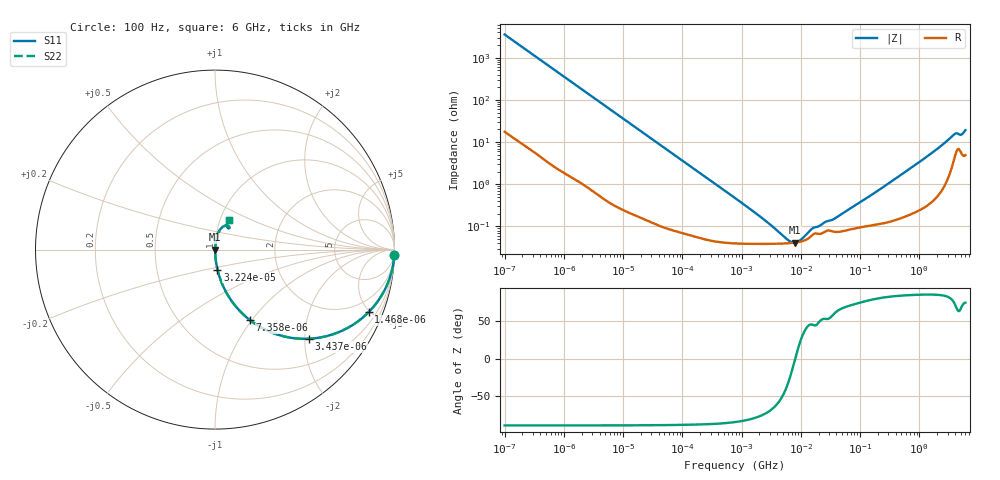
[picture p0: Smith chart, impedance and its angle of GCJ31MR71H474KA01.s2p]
!Murata Part Number: GCJ31MR71H474KA01
!These Parameters are Measured in Series Mode Connection
!Data Generated on Mar 13, 2026
!  o--ll--o
!Port1  Port2
!  o------o
!Operation Temp=25[degC], DC Bias Voltage=0[V]
!Freq. Start=100[Hz] Stop=6[GHz] 401[Steps]
# Hz S RI R 50
!Freq.(Hz) S11(Real) S11(Imag) S21(Real) S21(Imag) S12(Real) S12(Imag) S22(Real) S22(Imag)
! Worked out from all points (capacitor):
!   401 points, 100 Hz to 6 GHz, reference 50 ohm
!   read as one part in series: C = 447 nF near 109 Hz
!   lowest |Z| = 41.4 mohm at 7.948 MHz (marker M1)
!   series resonance near 8.045 MHz, so ESL is about 880 pH
!   S11 on the Smith chart (normalised r, x): 100 Hz: 1, -71; 1.468 kHz: 1.03, -4.89; 3.437 kHz: 1.01, -2.10; 7.358 kHz: 1.01, -0.98; 32.24 kHz: 1.00, -0.23; 6 GHz: 1.10, +0.37
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100  0.9991 -0.0281  0.000928 0.0281  0.000928 0.0281  0.9991 -0.0281
438  0.9846 -0.1206  0.0154 0.1206  0.0154 0.1206  0.9846 -0.1206
858  0.9448 -0.2259  0.0552 0.2259  0.0552 0.2259  0.9448 -0.2259
1468  0.8553 -0.349  0.1447 0.349  0.1447 0.349  0.8553 -0.349
2008  0.7607 -0.4238  0.2393 0.4238  0.2393 0.4238  0.7607 -0.4238
3437  0.5231 -0.4965  0.4769 0.4965  0.4769 0.4965  0.5231 -0.4965
7358  0.1954 -0.3934  0.8046 0.3934  0.8046 0.3934  0.1954 -0.3934
13772  0.0661 -0.2447  0.9339 0.2447  0.9339 0.2447  0.0661 -0.2447
32244  0.0137 -0.1109  0.9863 0.1109  0.9863 0.1109  0.0137 -0.1109
40335  0.00907 -0.0892  0.9909 0.0892  0.9909 0.0892  0.00907 -0.0892
774597  0.000418 -0.00471  0.9996 0.00471  0.9996 0.00471  0.000418 -0.00471
2372521  0.000388 -0.00142  0.9996 0.00142  0.9996 0.00142  0.000388 -0.00142
6075234  0.0004 -0.000263  0.9996 0.000263  0.9996 0.000263  0.0004 -0.000263
7947587  0.000414 -1.12e-05  0.9996 1.12e-05  0.9996 1.12e-05  0.000414 -1.12e-05
9941735  0.000437 0.000201  0.9996 -0.000201  0.9996 -0.000201  0.000437 0.000201
1.555665e7  0.00062 0.000637  0.9994 -0.000637  0.9994 -0.000637  0.00062 0.000637
3.80911e7  0.000743 0.00138  0.9993 -0.00138  0.9993 -0.00138  0.000743 0.00138
3.124326e8  0.0014 0.0107  0.9986 -0.0107  0.9986 -0.0107  0.0014 0.0107
1.369159e9  0.00522 0.0457  0.9948 -0.0457  0.9948 -0.0457  0.00522 0.0457
3.666503e9  0.0462 0.1288  0.9538 -0.1288  0.9538 -0.1288  0.0462 0.1288
5.016141e9  0.0703 0.1206  0.9297 -0.1206  0.9297 -0.1206  0.0703 0.1206
6e9  0.0757 0.1636  0.9243 -0.1636  0.9243 -0.1636  0.0757 0.1636
